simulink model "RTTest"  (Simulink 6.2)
settings: Solver=FixedStepDiscrete  StartTime=0.0  StopTime=inf  RelTol=1e-3
PreLoadFcn:
  | initialize
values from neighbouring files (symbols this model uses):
  nAct = 5    [Copy of initialize.m]    (also in initialize.m = 1)
  nAdcU = 6    [Copy of initialize.m]    (also in initialize.m = 5)
  nDout = 4    [Copy of initialize.m]    (also in initialize.m)
  nDucU = 2    [Copy of initialize.m]    (also in initialize.m)
  nEncU = 3    [Copy of initialize.m]    (also in initialize.m)
  node = completenodestruct(node)    [Copy of initialize.m]    (also in initialize.m)
libraries: xpclib x5

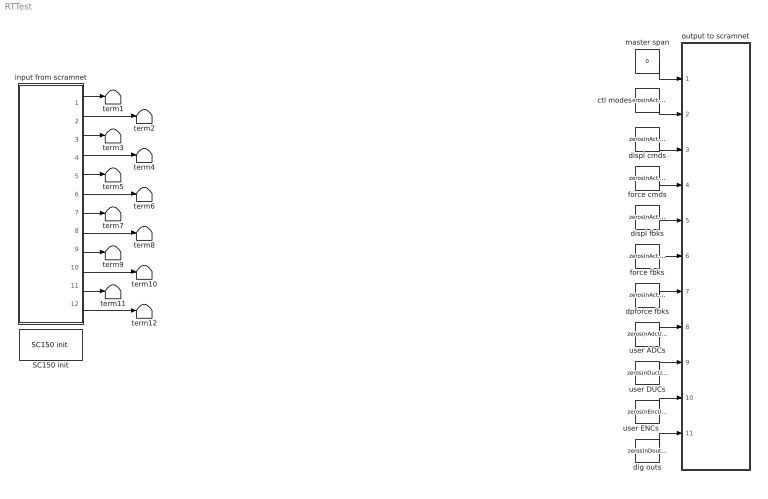
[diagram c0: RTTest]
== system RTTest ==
  SC150 init : xpclib/Shared Memory/Systran/SC150 init   node=node  pci=-1
  ctl modes : Constant  Value=zeros(nAct, 1)
  dig outs : Constant  Value=zeros(nDout, 1)  OutDataTypeMode=uint32
  displ cmds : Constant  Value=zeros(nAct, 1)
  displ fbks : Constant  Value=zeros(nAct, 1)
  dpforce fbks : Constant  Value=zeros(nAct, 1)
  force cmds : Constant  Value=zeros(nAct, 1)
  force fbks : Constant  Value=zeros(nAct, 1)
  input from scramnet : Subsystem
  master span : Constant  Value=0
  output to scramnet : Subsystem
  term{1..12} (12 alike) : Terminator
  user ADCs : Constant  Value=zeros(nAdcU, 1)
  user DUCs : Constant  Value=zeros(nDucU, 1)
  user ENCs : Constant  Value=zeros(nEncU, 1)
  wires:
  input from scramnet/6(force fbks) -> term6/1
  input from scramnet/10(user ducs) -> term10/1
  input from scramnet/12(dig inps) -> term12/1
  input from scramnet/4(force cmds) -> term4/1
  input from scramnet/5(displ fbks) -> term5/1
  input from scramnet/7(dpforce fbks) -> term7/1
  input from scramnet/9(user adcs) -> term9/1
  input from scramnet/11(user encs) -> term11/1
  input from scramnet/1(master span) -> term1/1
  input from scramnet/2(ctl modes) -> term2/1
  input from scramnet/3(displ cmds) -> term3/1
  master span/1 -> output to scramnet/1(master span)
  ctl modes/1 -> output to scramnet/2(ctl modes)
  displ cmds/1 -> output to scramnet/3(displ cmds)
  force cmds/1 -> output to scramnet/4(force cmds)
  user ADCs/1 -> output to scramnet/8(user adcs)
  user DUCs/1 -> output to scramnet/9(user ducs)
  user ENCs/1 -> output to scramnet/10(user encs)
  dig outs/1 -> output to scramnet/11(dig outs)
  displ fbks/1 -> output to scramnet/5(displ fbks)
  force fbks/1 -> output to scramnet/6(force fbks)
  dpforce fbks/1 -> output to scramnet/7(dpforce fbks)
  input from scramnet/8(valve cmds) -> term8/1

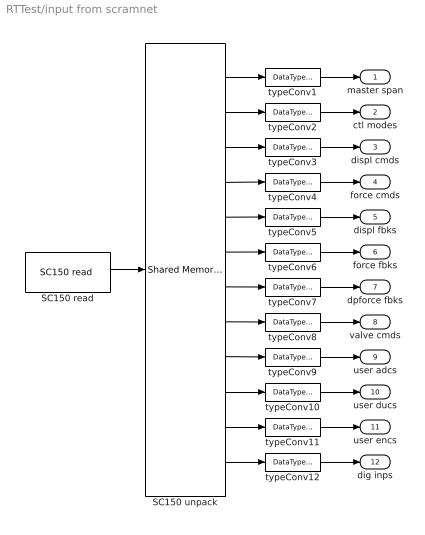
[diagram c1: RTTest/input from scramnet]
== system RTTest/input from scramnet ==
  SC150 read : xpclib/Shared Memory/Systran/SC150 read   partition=node.Partitions(12:23)  ts=samplePeriod  pci=-1
  SC150 unpack : xpclib/Shared Memory/Shared Memory Unpack   partition=node.Partitions(12:23)
  typeConv{1,3..11} (10 alike) : DataTypeConversion  OutDataTypeMode=double
  typeConv12 : DataTypeConversion  OutDataTypeMode=uint32
  typeConv2 : DataTypeConversion  OutDataTypeMode=uint32
  master span : Outport
  ctl modes : Outport  Port=2
  displ cmds : Outport  Port=3
  force cmds : Outport  Port=4
  displ fbks : Outport  Port=5
  force fbks : Outport  Port=6
  dpforce fbks : Outport  Port=7
  valve cmds : Outport  Port=8
  user adcs : Outport  Port=9
  user ducs : Outport  Port=10
  user encs : Outport  Port=11
  dig inps : Outport  Port=12
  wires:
  typeConv11/1 -> user encs/1
  typeConv10/1 -> user ducs/1
  typeConv12/1 -> dig inps/1
  typeConv9/1 -> user adcs/1
  typeConv8/1 -> valve cmds/1
  typeConv7/1 -> dpforce fbks/1
  typeConv6/1 -> force fbks/1
  typeConv5/1 -> displ fbks/1
  typeConv4/1 -> force cmds/1
  typeConv3/1 -> displ cmds/1
  typeConv1/1 -> master span/1
  SC150 read/1 -> SC150 unpack/1
  typeConv2/1 -> ctl modes/1
  SC150 unpack/1 -> typeConv1/1
  SC150 unpack/2 -> typeConv2/1
  SC150 unpack/3 -> typeConv3/1
  SC150 unpack/4 -> typeConv4/1
  SC150 unpack/5 -> typeConv5/1
  SC150 unpack/6 -> typeConv6/1
  SC150 unpack/7 -> typeConv7/1
  SC150 unpack/8 -> typeConv8/1
  SC150 unpack/9 -> typeConv9/1
  SC150 unpack/10 -> typeConv10/1
  SC150 unpack/11 -> typeConv11/1
  SC150 unpack/12 -> typeConv12/1

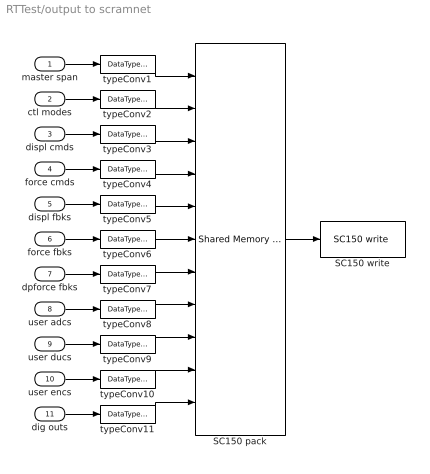
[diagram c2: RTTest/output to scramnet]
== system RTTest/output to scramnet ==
  master span : Inport  Port=1  LatchInput=off
  ctl modes : Inport  Port=2  LatchInput=off
  displ cmds : Inport  Port=3  LatchInput=off
  force cmds : Inport  Port=4  LatchInput=off
  displ fbks : Inport  Port=5  LatchInput=off
  force fbks : Inport  Port=6  LatchInput=off
  dpforce fbks : Inport  Port=7  LatchInput=off
  user adcs : Inport  Port=8  LatchInput=off
  user ducs : Inport  Port=9  LatchInput=off
  user encs : Inport  Port=10  LatchInput=off
  dig outs : Inport  Port=11  LatchInput=off
  SC150 pack : xpclib/Shared Memory/Shared Memory Pack   partition=node.Partitions(1:11)
  SC150 write : xpclib/Shared Memory/Systran/SC150 write   partition=node.Partitions(1:11)  ts=samplePeriod  pci=-1
  typeConv{1,3..10} (9 alike) : DataTypeConversion  OutDataTypeMode=single
  typeConv11 : DataTypeConversion  OutDataTypeMode=uint32
  typeConv2 : DataTypeConversion  OutDataTypeMode=uint32
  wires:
  typeConv11/1 -> SC150 pack/11
  typeConv10/1 -> SC150 pack/10
  typeConv9/1 -> SC150 pack/9
  typeConv8/1 -> SC150 pack/8
  typeConv7/1 -> SC150 pack/7
  typeConv6/1 -> SC150 pack/6
  typeConv5/1 -> SC150 pack/5
  dig outs/1 -> typeConv11/1
  user encs/1 -> typeConv10/1
  user ducs/1 -> typeConv9/1
  user adcs/1 -> typeConv8/1
  dpforce fbks/1 -> typeConv7/1
  force fbks/1 -> typeConv6/1
  displ fbks/1 -> typeConv5/1
  force cmds/1 -> typeConv4/1
  master span/1 -> typeConv1/1
  SC150 pack/1 -> SC150 write/1
  displ cmds/1 -> typeConv3/1
  ctl modes/1 -> typeConv2/1
  typeConv1/1 -> SC150 pack/1
  typeConv2/1 -> SC150 pack/2
  typeConv3/1 -> SC150 pack/3
  typeConv4/1 -> SC150 pack/4
